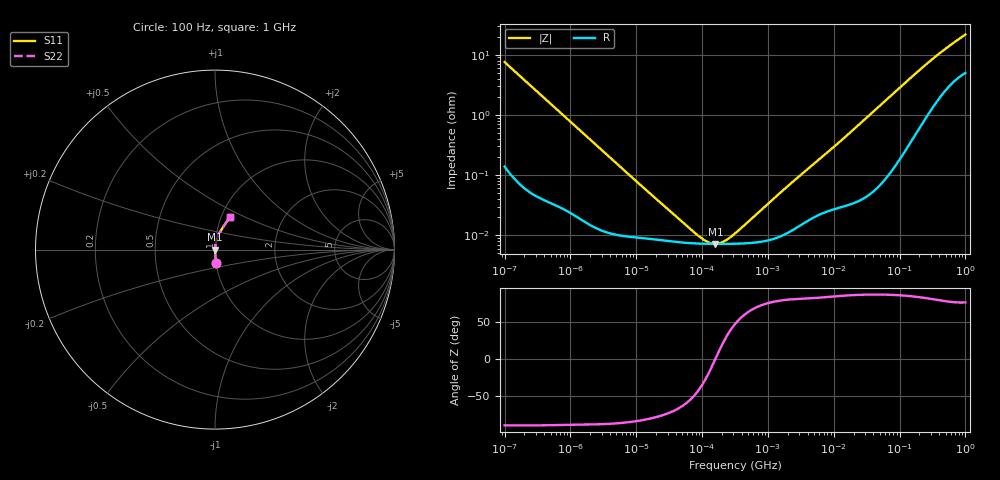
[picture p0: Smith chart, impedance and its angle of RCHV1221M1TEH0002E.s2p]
! RCHV1221M1TEH0002E  S-PARAMETER MODEL  (AEC-Q200 qualified)
! Model Generated by ELNA Corporation (http://www.ty-top.com)
! Version 1.0
! ELNA Control No. 240229
! Copyright (c) 2024 ELNA CO.,LTD. All Rights Reserved.
! Products Name : CONDUCTIVE POLYMER HYBRID ALUMINUM ELECTROLYTIC CAPACITORS
! Characteristics :
!  Capacitance  :  220uF  ,  Rated voltage  :  25V
!  Operating Temp. Range  :  -55 to +105 degC  ,  Endurance  :  10000hr at 105 degC
!  Dimension D  :  8mm  ,  Dimension L  :  10mm
! Frequency Range : 100Hz - 1GHz
! External Node Assignments :
!  1  o---| |---o  2
# MHz S RI R 50
!Freq[MHz].  S11 Real  S11 Imag  S21 Real  S21 Imag  S12 Real  S12 Imag  S22 Real  S22 Imag
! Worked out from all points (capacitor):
!   401 points, 100 Hz to 1 GHz, reference 50 ohm
!   read as one part in series: C = 211 uF near 108 Hz
!   lowest |Z| = 7.17 mohm at 159.4 kHz (marker M1)
!   series resonance near 158.2 kHz, so ESL is about 4.8 nH
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0.0001  0.00701 -0.0748  0.993 0.0748  0.993 0.0748  0.00701 -0.0748
0.000113  0.00559 -0.0664  0.9944 0.0664  0.9944 0.0664  0.00559 -0.0664
0.000183  0.00235 -0.0411  0.9977 0.0411  0.9977 0.0411  0.00235 -0.0411
0.000309  0.00104 -0.0244  0.999 0.0244  0.999 0.0244  0.00104 -0.0244
0.001488  0.000206 -0.00519  0.9998 0.00519  0.9998 0.00519  0.000206 -0.00519
0.022131  8.37e-05 -0.000355  0.9999 0.000355  0.9999 0.000355  8.37e-05 -0.000355
0.080353  7.3e-05 -7.65e-05  0.9999 7.65e-05  0.9999 7.65e-05  7.3e-05 -7.65e-05
0.087096  7.27e-05 -6.63e-05  0.9999 6.63e-05  0.9999 6.63e-05  7.27e-05 -6.63e-05
0.094406  7.25e-05 -5.66e-05  0.9999 5.66e-05  0.9999 5.66e-05  7.25e-05 -5.66e-05
0.159404  7.17e-05 7.94e-07  0.9999 -7.94e-07  0.9999 -7.94e-07  7.17e-05 7.94e-07
0.269153  7.19e-05 5.86e-05  0.9999 -5.86e-05  0.9999 -5.86e-05  7.19e-05 5.86e-05
0.291743  7.2e-05 6.85e-05  0.9999 -6.85e-05  0.9999 -6.85e-05  7.2e-05 6.85e-05
0.316228  7.22e-05 7.88e-05  0.9999 -7.88e-05  0.9999 -7.88e-05  7.22e-05 7.88e-05
1.788546  0.000103 0.000578  0.9999 -0.000578  0.9999 -0.000578  0.000103 0.000578
4.704354  0.000193 0.00144  0.9998 -0.00144  0.9998 -0.00144  0.000193 0.00144
13.96368  0.000315 0.00401  0.9997 -0.00401  0.9997 -0.00401  0.000315 0.00401
69.9842  0.00143 0.0197  0.9986 -0.0197  0.9986 -0.0197  0.00143 0.0197
156.6751  0.00575 0.0431  0.9942 -0.0431  0.9942 -0.0431  0.00575 0.0431
323.5937  0.0203 0.0825  0.9797 -0.0825  0.9797 -0.0825  0.0203 0.0825
568.8529  0.0458 0.1265  0.9542 -0.1265  0.9542 -0.1265  0.0458 0.1265
922.5714  0.078 0.1745  0.922 -0.1745  0.922 -0.1745  0.078 0.1745
1000  0.0844 0.1841  0.9156 -0.1841  0.9156 -0.1841  0.0844 0.1841
